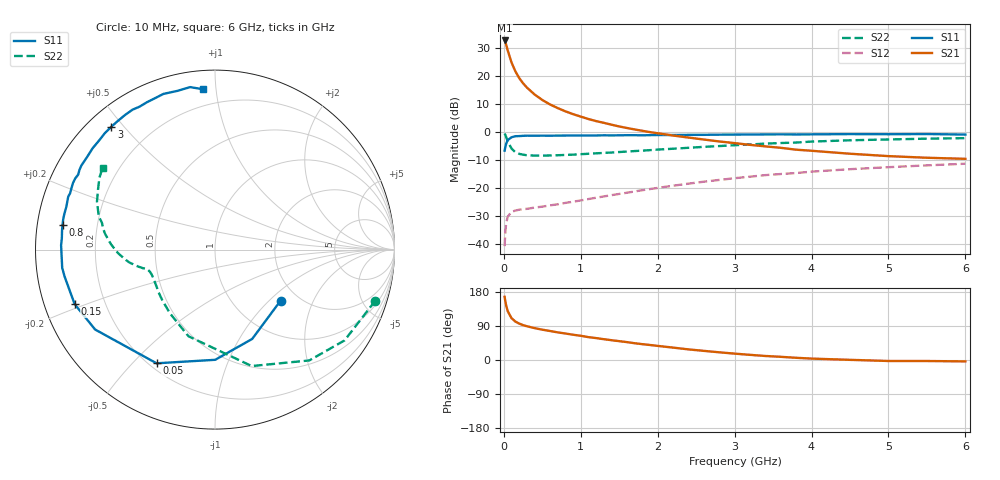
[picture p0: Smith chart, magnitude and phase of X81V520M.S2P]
! SIEMENS Small Signal Semiconductors
! BFP136W
! Si NPN RF Bipolar Junction Transistor in SOT343
! VCE = 1.5 V  IC = 20 mA
! Common Emitter S-Parameters:  September  1994
# GHz  S  MA  R  50
!  f  S11  S21  S12  S22
! GHz  MAG  ANG  MAG  ANG  MAG  ANG  MAG  ANG
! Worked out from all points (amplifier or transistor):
!   40 points, 10 MHz to 6 GHz, reference 50 ohm
!   highest |S21| = 32.5 dB at 10 MHz (marker M1)
!   |S21| within 3 dB of that: start of sweep to 45.27 MHz
!   unconditionally stable (mu >= 1): 831.7 MHz to 2.808 GHz; 5.94 GHz to end of sweep
!   at 200 MHz: K = 0.34, MSG = 23.4 dB, |S12| = -27.7 dB
!   at 1.5 GHz: K = 1.17, MAG = 9.5 dB, |S12| = -22.1 dB
!   at 6 GHz: K = 1.01, MAG = 0.3 dB, |S12| = -11.3 dB
!   S11 on the Smith chart (normalised r, x): 10 MHz: 1.62, -1.18; 50 MHz: 0.23, -0.59; 150 MHz: 0.09, -0.19; 800 MHz: 0.08, +0.08; 3 GHz: 0.07, +0.46; 6 GHz: 0.10, +0.92
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0.01  0.4632 -37.9  42.23 166.8  0.0093 75.7  0.9373 -17.7
0.02  0.5391 -67.4  38.99 154.4  0.0171 65.6  0.8816 -35.0
0.03  0.614 -89.9  35.7 144.2  0.0235 56.5  0.8109 -49.6
0.05  0.7122 -117.2  28.3 129.0  0.0311 42.6  0.6803 -72.5
0.1  0.8027 -146.3  17.12 110.3  0.0378 28.7  0.505 -107.0
0.15  0.8389 -158.7  11.94 101.4  0.04 24.9  0.4352 -125.1
0.2  0.8424 -165.3  9.045 96.0  0.0414 23.2  0.4072 -136.2
0.25  0.8514 -169.9  7.32 92.0  0.0424 23.0  0.3936 -143.3
0.3  0.8574 -173.2  6.135 89.1  0.0428 23.8  0.3845 -148.2
0.4  0.8555 -178.4  4.627 84.1  0.0452 26.5  0.3792 -154.4
0.5  0.8579 178.3  3.694 80.0  0.0469 29.0  0.3789 -158.2
0.6  0.8557 175.7  3.077 76.6  0.0494 32.1  0.3813 -160.4
0.7  0.8591 172.7  2.651 72.9  0.0516 35.0  0.3848 -161.8
0.8  0.8608 170.7  2.321 69.9  0.0547 37.0  0.3895 -163.0
1.1  0.8619 164.0  1.692 60.3  0.064 43.1  0.4083 -165.1
1.6  0.8739 154.9  1.173 47.2  0.0829 48.9  0.4472 -168.4
2.2  0.8797 144.3  0.862 32.7  0.1105 50.7  0.5019 -173.6
3  0.8957 130.1  0.632 16.8  0.1503 47.3  0.58 177.1
3.2  0.8984 126.9  0.588 13.6  0.1599 45.9  0.5983 174.5
4.5  0.9137 108.3  0.409 0.4  0.2173 34.7  0.7093 158.0
5.5  0.9159 98.7  0.347 -2.7  0.2541 26.4  0.7583 148.1
6  0.8964 94.4  0.332 -3.7  0.2718 21.8  0.7746 144.0
